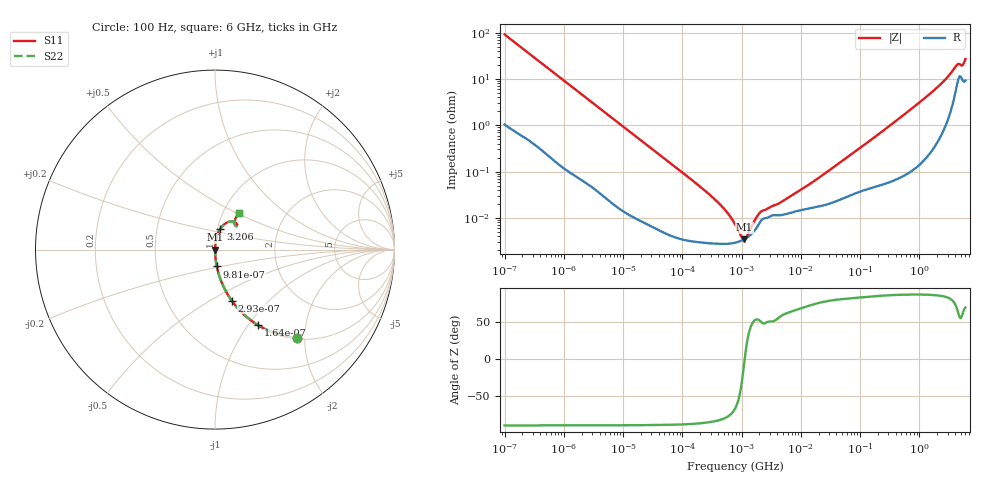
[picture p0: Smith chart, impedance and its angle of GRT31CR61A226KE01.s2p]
!Murata Part Number: GRT31CR61A226KE01
!These Parameters are Measured in Series Mode Connection
!Data Generated on Jun 19, 2026
!  o--ll--o
!Port1  Port2
!  o------o
!Operation Temp=25[degC], DC Bias Voltage=0[V]
!Freq. Start=100[Hz] Stop=6[GHz] 401[Steps]
# Hz S RI R 50
!Freq.(Hz) S11(Real) S11(Imag) S21(Real) S21(Imag) S12(Real) S12(Imag) S22(Real) S22(Imag)
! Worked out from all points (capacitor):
!   401 points, 100 Hz to 6 GHz, reference 50 ohm
!   read as one part in series: C = 17.4 uF near 109 Hz
!   lowest |Z| = 3.46 mohm at 1.108 MHz (marker M1)
!   series resonance near 1.129 MHz, so ESL is about 1.1 nH
!   S11 on the Smith chart (normalised r, x): 100 Hz: 1.02, -1.83; 164 Hz: 1.01, -1.12; 293 Hz: 1.01, -0.63; 981 Hz: 1.00, -0.19; 3.206 GHz: 1.03, +0.24; 6 GHz: 1.18, +0.51
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100  0.4553 -0.4924  0.5447 0.4924  0.5447 0.4924  0.4553 -0.4924
164  0.2414 -0.4219  0.7586 0.4219  0.7586 0.4219  0.2414 -0.4219
293  0.0931 -0.284  0.9069 0.284  0.9069 0.284  0.0931 -0.284
524  0.0323 -0.1705  0.9677 0.1705  0.9677 0.1705  0.0323 -0.1705
981  0.0101 -0.0937  0.9899 0.0937  0.9899 0.0937  0.0101 -0.0937
2008  0.00281 -0.0464  0.9972 0.0464  0.9972 0.0464  0.00281 -0.0464
40335  5.94e-05 -0.00238  0.9999 0.00238  0.9999 0.00238  5.94e-05 -0.00238
276587  2.85e-05 -0.000331  1 0.000331  1 0.000331  2.85e-05 -0.000331
432798  2.74e-05 -0.000193  1 0.000193  1 0.000193  2.74e-05 -0.000193
647581  2.79e-05 -0.000102  1 0.000102  1 0.000102  2.79e-05 -0.000102
774597  2.9e-05 -6.75e-05  1 6.75e-05  1 6.75e-05  2.9e-05 -6.75e-05
1108252  3.45e-05 -3.2e-06  1 3.2e-06  1 3.2e-06  3.45e-05 -3.2e-06
1734173  5.75e-05 7.76e-05  0.9999 -7.76e-05  0.9999 -7.76e-05  5.75e-05 7.76e-05
2169299  8.96e-05 0.000107  0.9999 -0.000107  0.9999 -0.000107  8.96e-05 0.000107
4440638  0.000114 0.000178  0.9999 -0.000178  0.9999 -0.000178  0.000114 0.000178
1.555665e7  0.000165 0.000561  0.9998 -0.000561  0.9998 -0.000561  0.000165 0.000561
3.124326e8  0.000679 0.00962  0.9993 -0.00962  0.9993 -0.00962  0.000679 0.00962
1.497423e9  0.00464 0.0469  0.9954 -0.0469  0.9954 -0.0469  0.00464 0.0469
3.205649e9  0.0293 0.115  0.9707 -0.115  0.9707 -0.115  0.0293 0.115
4.193612e9  0.0848 0.1566  0.9152 -0.1566  0.9152 -0.1566  0.0848 0.1566
5.245841e9  0.1121 0.1339  0.8879 -0.1339  0.8879 -0.1339  0.1121 0.1339
6e9  0.1313 0.2013  0.8687 -0.2013  0.8687 -0.2013  0.1313 0.2013
